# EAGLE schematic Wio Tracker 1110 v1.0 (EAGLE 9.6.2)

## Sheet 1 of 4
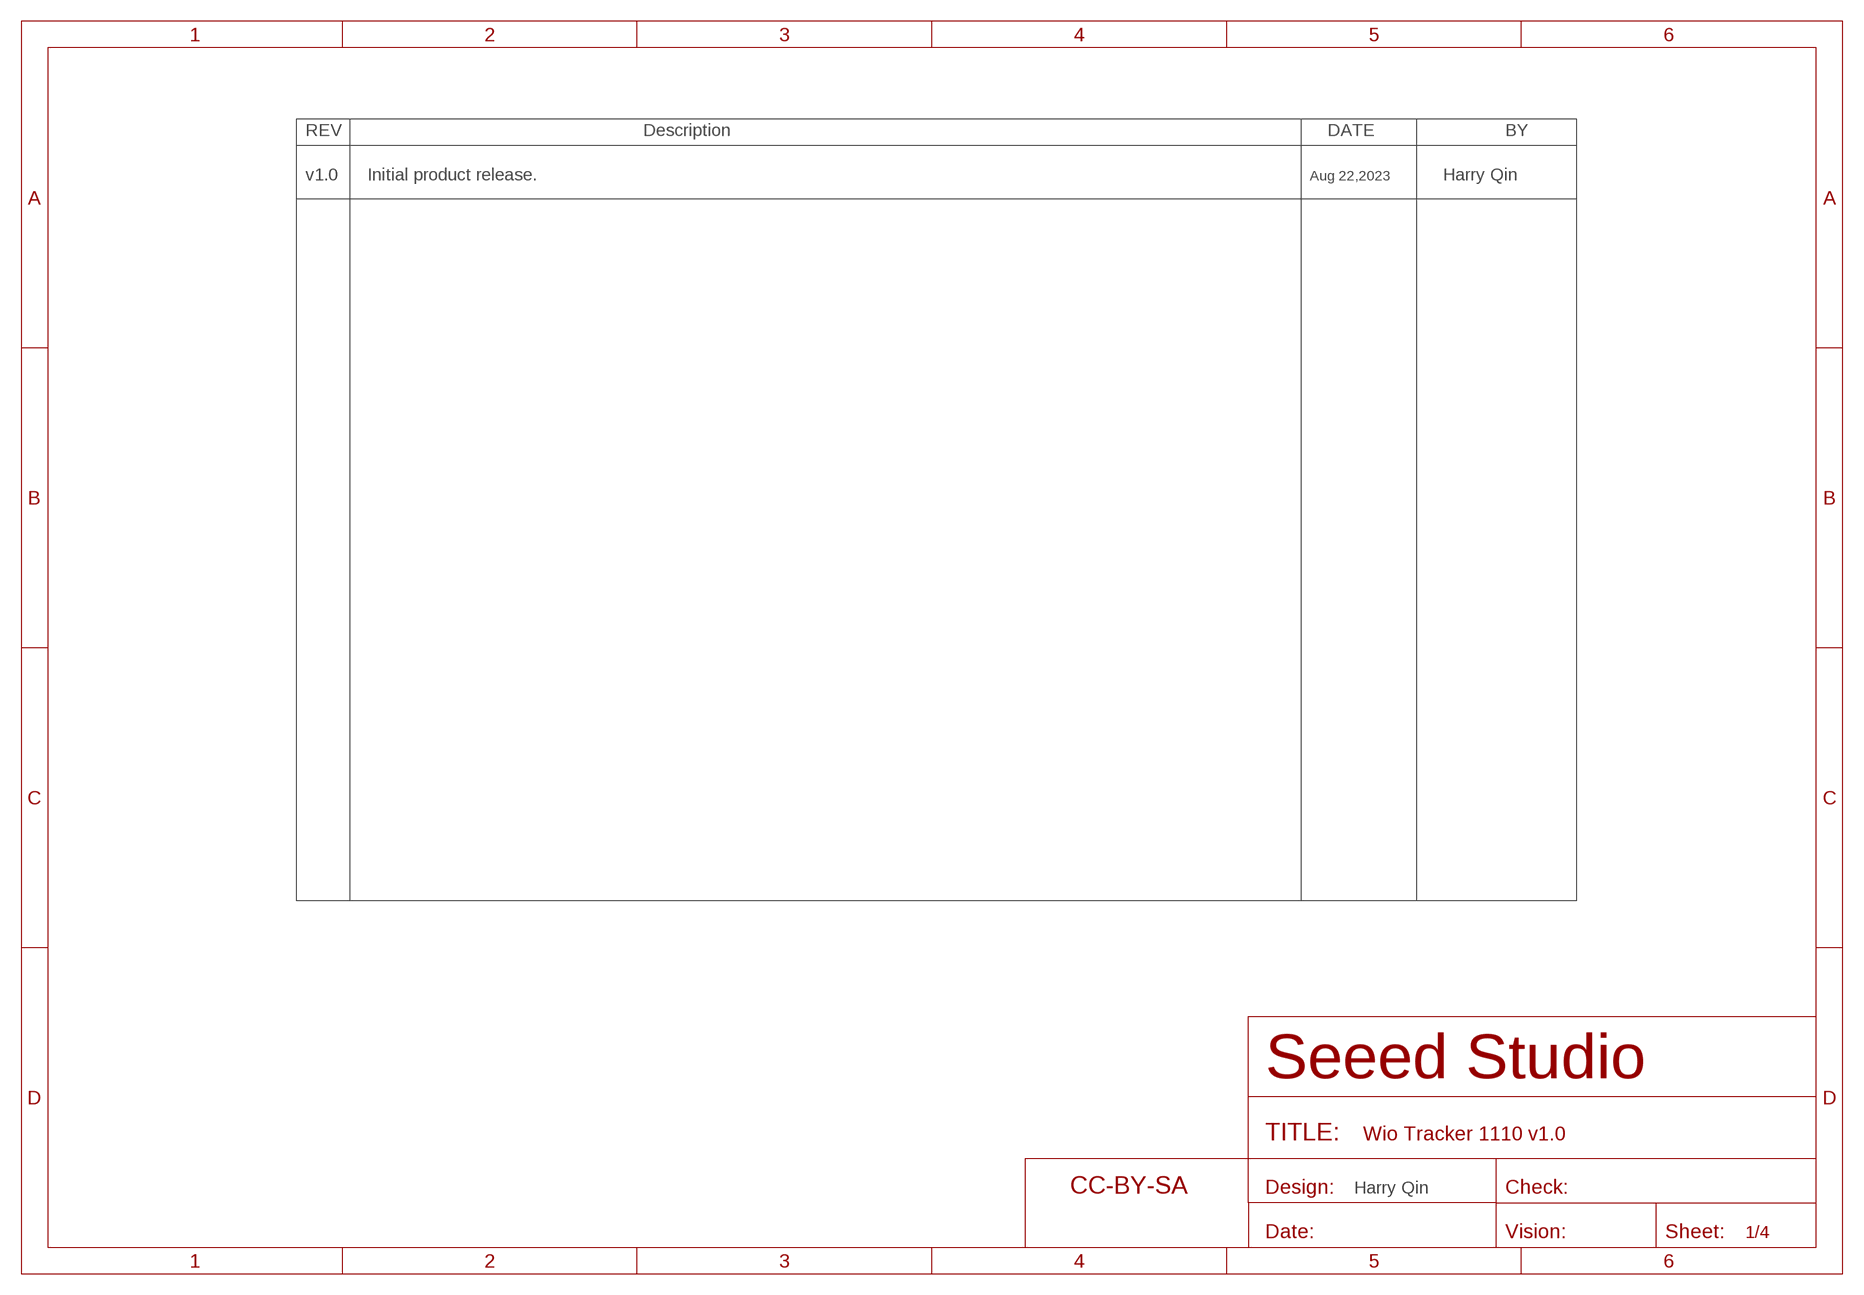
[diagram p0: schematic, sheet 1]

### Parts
FR2  SEEEDSTUDIO-OPEN-SCH-FRAME  [SEEEDSTUDIO-PCB-FRAME]

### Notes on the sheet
- v1.0 | Initial product release. | Aug 22,2023 | Harry Qin
- Harry Qin

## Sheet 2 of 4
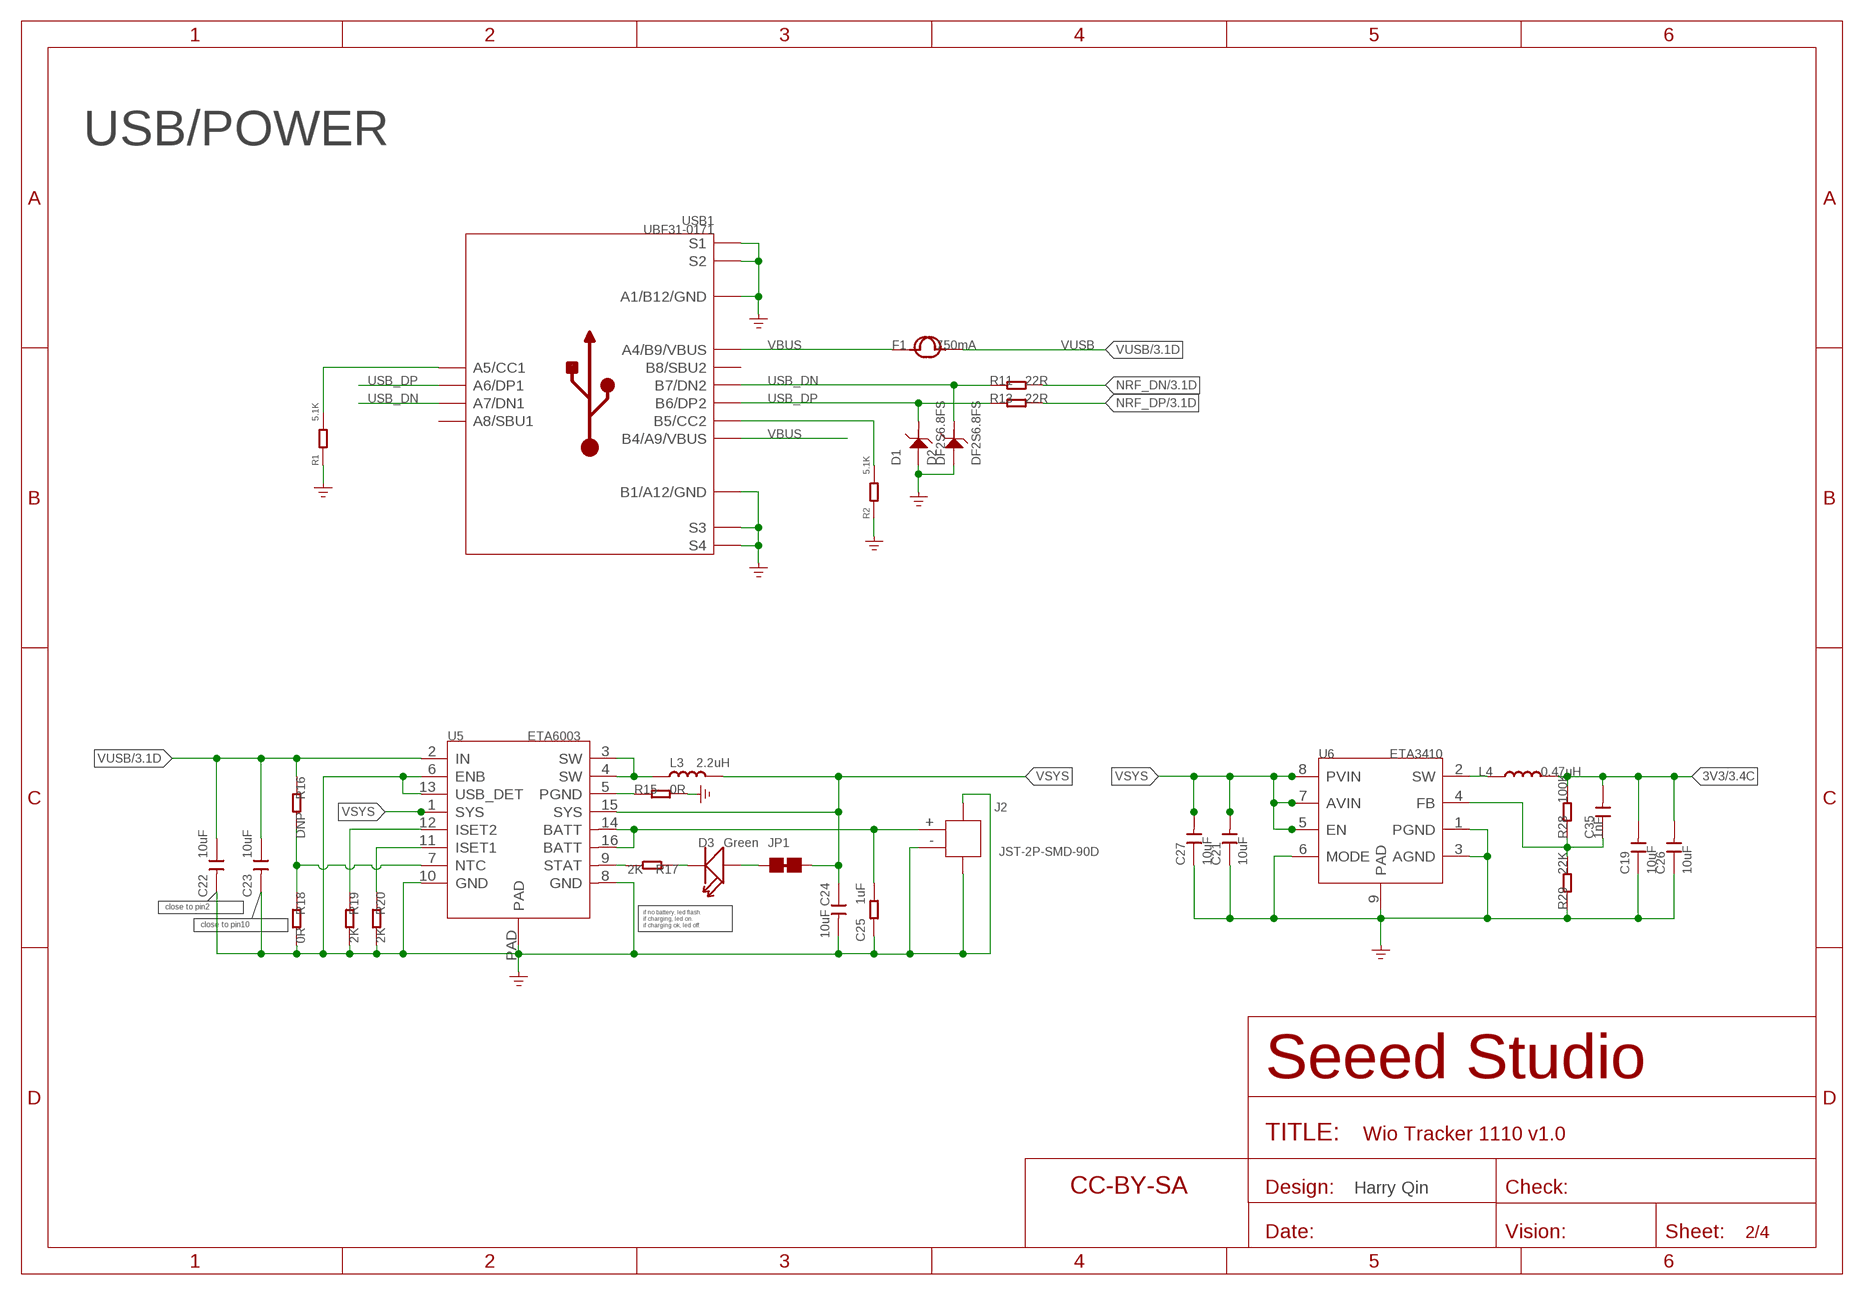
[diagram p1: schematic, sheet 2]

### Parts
C19  10uF  CAP-0603  [C0603]
C21  10uF  CAP-0603  [C0603]
C22  10uF  CAP-0805  [C0805]
C23  10uF  CAP-0805  [C0805]
C24  10uF  CAP-0805  [C0805]
C25  1uF  RES-0402  [R0402]
C26  10uF  CAP-0603  [C0603]
C27  10uF  CAP-0603  [C0603]
C35  1nF  CAP-0402  [C0402]
D1  DF2S6.8FS  D-ESD-2P'DF2S6.8FS'  [SOD-923]
D2  DF2S6.8FS  D-ESD-2P'DF2S6.8FS'  [SOD-923]
D3  Green  LED-0402  [LED-0402]
F1  750mA  FUSE+'1206'  [FS1206]
FR1  SEEEDSTUDIO-OPEN-SCH-FRAME  [SEEEDSTUDIO-PCB-FRAME]
J2  JST-2P-SMD-90D  JST-2P-SMD'2.0'  [HW2-SMD-2.0-90D]
JP1  JP-2P-SHORT'1'  [2P-SMD-SHORT]
L3  2.2uH  INDUCTOR'0806'  [L0806]
L4  0.47uH  L-MPM201610SR33_T  [L201610@1]
R1  5.1K  RES-0402  [R0402]
R2  5.1K  RES-0402  [R0402]
R11  22R  RES-0402  [R0402]
R13  22R  RES-0402  [R0402]
R15  0R  RES-0402  [R0402]
R16  DNP  RES-0402  [R0402]
R17  2K  RES-0402  [R0402]
R18  0R  RES-0402  [R0402]
R19  2K  RES-0402  [R0402]
R20  2K  RES-0402  [R0402]
R28  100K  RES-0402  [R0402]
R29  22K  RES-0402  [R0402]
U5  ETA6003  PMIC-ETA6003  [QFN16G-0.5-3X3MM]
U6  ETA3410  CONVERTER-ETA3410  [DFN8G-0.5-2X2MM]
USB1  UBF31-0171  USB2.0-TYPE-C-320010698  [USB2.0-TYPE-C]

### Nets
3V3: C19.2 C26.2 C35.2 L4.2 R28.2 ; also sheet 3,4
GND: C19.1 C21.1 C22.2 C23.2 C24.2 C25.2 C26.1 C27.1 D1.2 D2.2 J2.3 J2.4 J2.- R1.1 R2.1 R15.2 R18.2 R19.2 R20.2 R29.1 U5.6(ENB) U5.8(GND) U5.10(GND) U5.13(USB_DET) U5.PAD U6.1(PGND) U6.3(AGND) U6.6(MODE) U6.9(PAD) USB1.A1_B12(A1/B12/GND) USB1.B1_A12(B1/A12/GND) USB1.S1 USB1.S2 USB1.S3 USB1.S4 USB1.S5(S1) USB1.S6(S2) ; supply symbol labelled GND_POWER ; also sheet 3,4
N$1: R1.2 USB1.A5(A5/CC1)
N$2: R2.2 USB1.B5(B5/CC2)
N$10: D3.+ JP1.1
N$26: L3.1 U5.3(SW) U5.4(SW)
N$28: C25.1 J2.+ U5.14(BATT) U5.16(BATT)
N$29: L4.1 U6.2(SW)
N$30: D3.- R17.1
N$31: R17.2 U5.9(STAT)
N$32: C35.1 R28.1 R29.2 U6.4(FB)
N$33: R16.2 R18.1 U5.7(NTC)
N$34: R20.1 U5.11(ISET1)
N$36: R19.1 U5.12(ISET2)
N$37: R15.1 U5.5(PGND)
NRF_DN: R11.2 ; also sheet 3
NRF_DP: R13.2 ; also sheet 3
USB_DN: D2.1 R11.1 USB1.A7(A7/DN1) USB1.B7(B7/DN2)
USB_DP: D1.1 R13.1 USB1.A6(A6/DP1) USB1.B6(B6/DP2)
VBUS: F1.1 USB1.A4_B9(A4/B9/VBUS) USB1.B4_A9(B4/A9/VBUS)
VSYS: C21.2 C24.1 C27.2 JP1.2 L3.2 U5.1(SYS) U5.15(SYS) U6.5(EN) U6.7(AVIN) U6.8(PVIN)
VUSB: C22.1 C23.1 F1.2 R16.1 U5.2(IN) ; also sheet 3
Unconnected: USB1.A8(A8/SBU1) USB1.B8(B8/SBU2)

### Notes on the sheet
- USB/POWER
- close to pin2
- close to pin10
- if no battery, led flash.
  if charging, led on.
  if charging ok, led off.
- Harry Qin

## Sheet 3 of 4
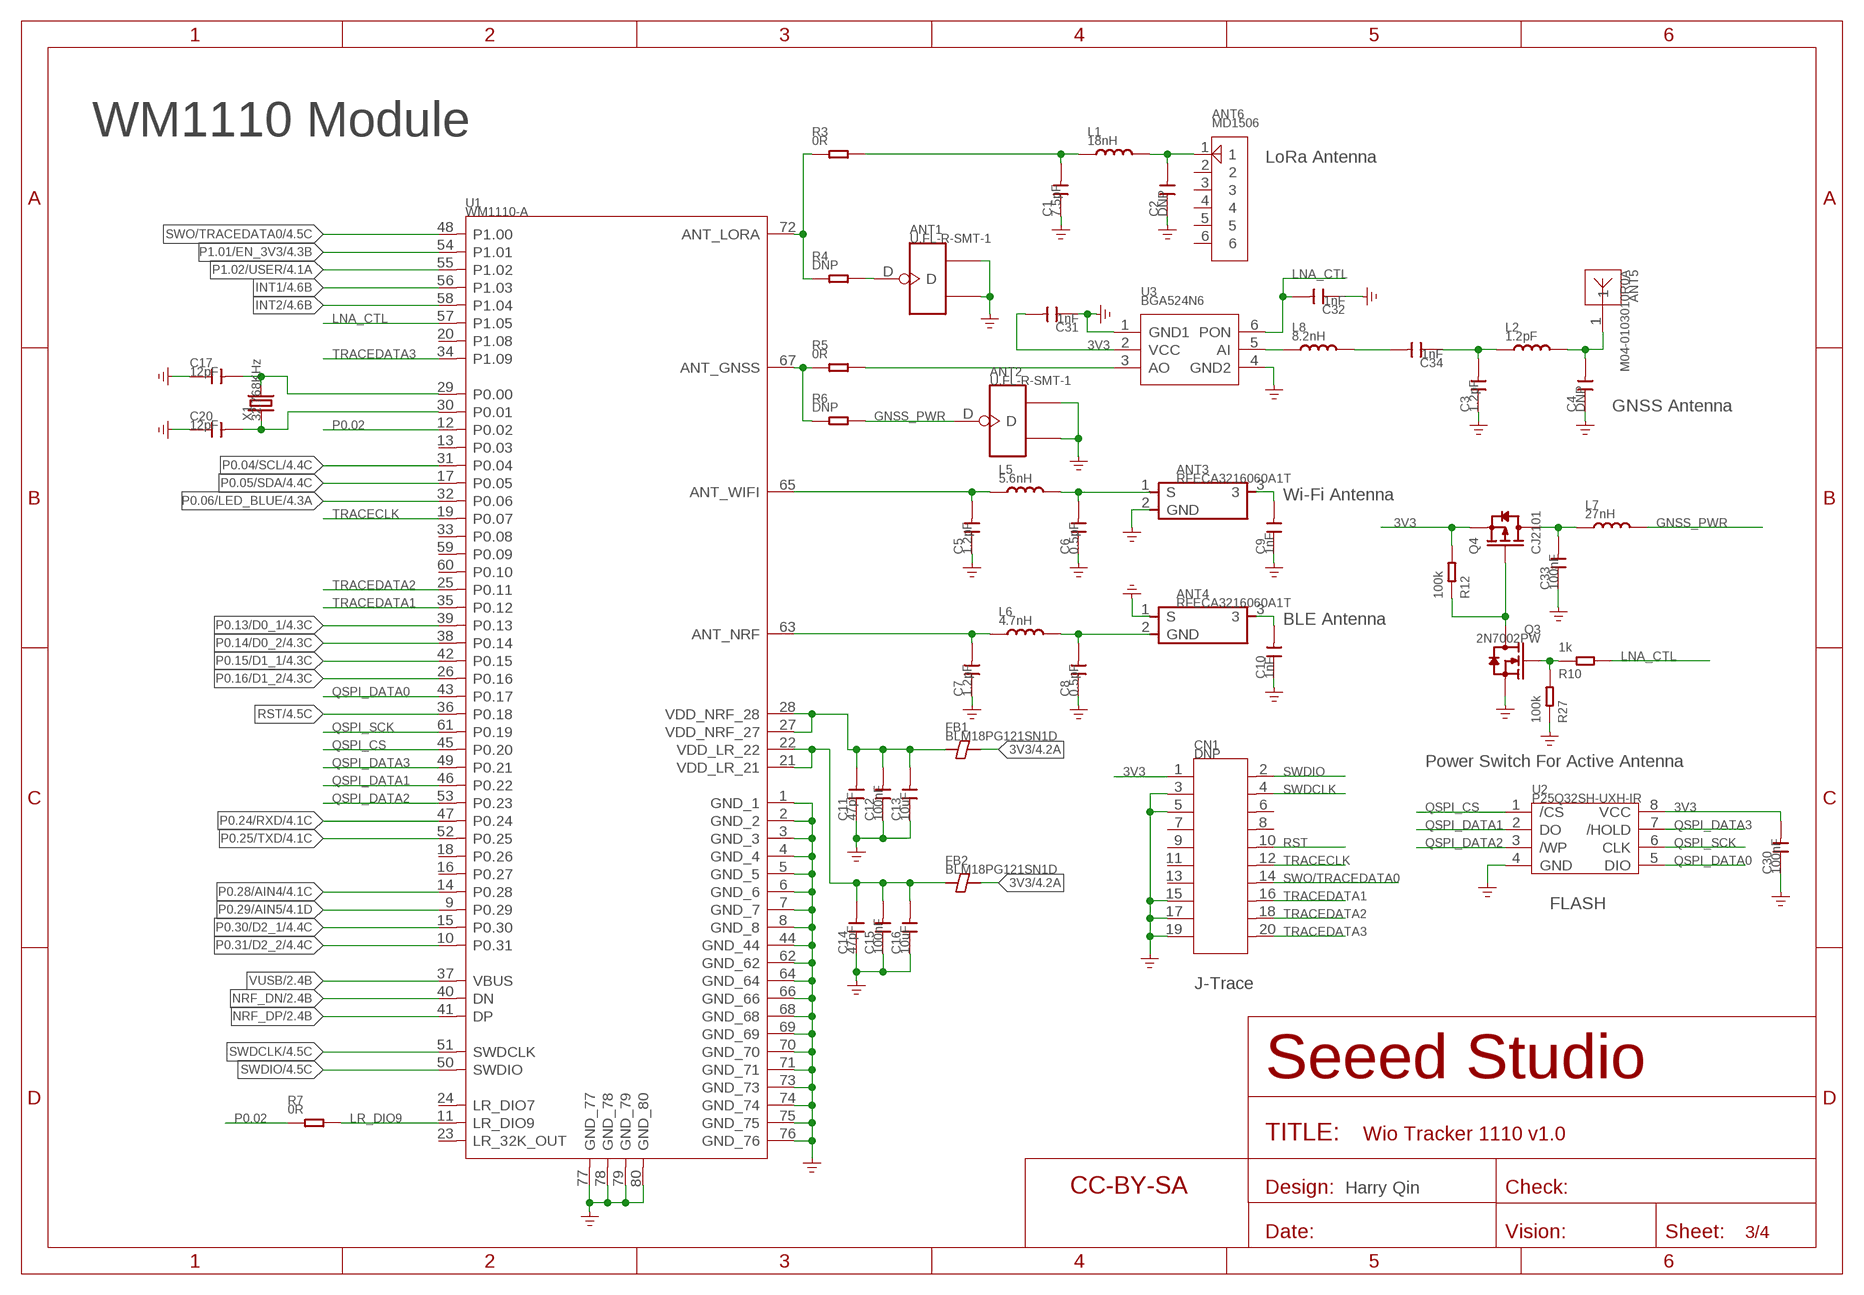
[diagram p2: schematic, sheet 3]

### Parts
ANT1  U.FL-R-SMT-1  ANTENNA-U-FL-320110048  [U-FL3P-SMD-2.6X2.6X1.0MM]
ANT2  U.FL-R-SMT-1  ANTENNA-U-FL-320110048  [U-FL3P-SMD-2.6X2.6X1.0MM]
ANT3  RFECA3216060A1T  ANTENNA-AN3116  [ANT-SMD3P-3.1X1.6X1.04MM]
ANT4  RFECA3216060A1T  ANTENNA-AN3116  [ANT-SMD3P-3.1X1.6X1.04MM]
ANT5  M04-0103010R0A  ANTENNA-M04-0103010R0A  [ANT-DIP-14X6X4MM]
ANT6  MD1506  ANTENNA-MD1506-12N  [ANT6-SMD-15X6.5X1.63MM]
C1  7.5pF  CAP-0402  [C0402]
C2  DNP  CAP-0402  [C0402]
C3  1.2pF  CAP-0402  [C0402]
C4  DNP  CAP-0402  [C0402]
C5  1.2pF  CAP-0402  [C0402]
C6  0.5pF  CAP-0402  [C0402]
C7  1.2pF  CAP-0402  [C0402]
C8  0.5pF  CAP-0402  [C0402]
C9  1nF  CAP-0402  [C0402]
C10  1nF  CAP-0402  [C0402]
C11  47pF  CAP-0402  [C0402]
C12  100nF  CAP-0402  [C0402]
C13  10uF  CAP-0603  [C0603]
C14  47pF  CAP-0402  [C0402]
C15  100nF  CAP-0402  [C0402]
C16  10uF  CAP-0603  [C0603]
C17  12pF  CAP-0402  [C0402]
C20  12pF  CAP-0402  [C0402]
C30  100nF  CAP-0402  [C0402]
C31  1nF  CAP-0402  [C0402]
C32  1nF  CAP-0402  [C0402]
C33  100nF  CAP-0402  [C0402]
C34  1nF  CAP-0402  [C0402]
CN1  DNP  HEADER-2X10P-1/3-1.27  [H2X10-1.27-12.7X3X5.7MM]
FB1  BLM18PG121SN1D  FERRITE-BEAD-0603  [F0603]
FB2  BLM18PG121SN1D  FERRITE-BEAD-0603  [F0603]
FR3  SEEEDSTUDIO-OPEN-SCH-FRAME  [SEEEDSTUDIO-PCB-FRAME]
L1  18nH  INDUCTOR'0402'  [L0402]
L2  1.2pF  INDUCTOR'0402'  [L0402]
L5  5.6nH  INDUCTOR'0402'  [L0402]
L6  4.7nH  INDUCTOR'0402'  [L0402]
L7  27nH  INDUCTOR'0402'  [L0402]
L8  8.2nH  INDUCTOR'0402'  [L0402]
Q3  2N7002PW  MOSFET-N-SI1304BDL  [SOT-323]
Q4  CJ2101  MOSFET-P-SOT323  [SOT-323]
R3  0R  RES-0402  [R0402]
R4  DNP  RES-0402  [R0402]
R5  0R  RES-0402  [R0402]
R6  DNP  RES-0402  [R0402]
R7  0R  RES-0402  [R0402]
R10  1k  RES-0402  [R0402]
R12  100k  RES-0402  [R0402]
R27  100k  RES-0402  [R0402]
U1  WM1110-A  MODULE-LORAMODULE  [MODULE72_0D9_20X20X2MM]
U2  P25Q32SH-UXH-IR  FLASH-W25X80-FZUIH1  [USON8-0.5-3X2MM]
U3  BGA524N6  GNSS-BGA524N6  [BGA6-0.4-1.1X0.7X0.4MM]
X1  32.768KHz  CRYSTAL-2P'NX2012SA'  [X2-SMD-L2.0X1.2X0.55MM]

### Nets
3V3: C30.2 C31.2 CN1.1 FB1.2 FB2.2 Q4.2(S) R12.2 U2.8(VCC) U3.2(VCC) ; also sheet 2,4
GND: ANT1.GND1 ANT1.GND2 ANT2.GND1 ANT2.GND2 ANT3.2(GND) ANT4.1(S) C1.1 C2.1 C3.1 C4.1 C5.1 C6.1 C7.1 C8.1 C9.1 C10.1 C11.1 C12.1 C13.1 C14.1 C15.1 C16.1 C17.1 C20.1 C30.1 C31.1 C32.1 C33.1 CN1.3 CN1.5 CN1.15 CN1.17 CN1.19 Q3.2(S) R27.1 U1.1(GND_1) U1.2(GND_2) U1.3(GND_3) U1.4(GND_4) U1.5(GND_5) U1.6(GND_6) U1.7(GND_7) U1.8(GND_8) U1.44(GND_44) U1.62(GND_62) U1.64(GND_64) U1.66(GND_66) U1.68(GND_68) U1.69(GND_69) U1.70(GND_70) U1.71(GND_71) U1.73(GND_73) U1.74(GND_74) U1.75(GND_75) U1.76(GND_76) U1.77(GND_77) U1.78(GND_78) U1.79(GND_79) U1.80(GND_80) U2.4(GND) U3.1(GND1) U3.4(GND2) ; supply symbol labelled GND_POWER ; also sheet 2,4
GNSS_PWR: ANT2.D L7.2 R6.2
INT1: U1.56(P1.03) ; also sheet 4
INT2: U1.58(P1.04) ; also sheet 4
LNA_CTL: C32.2 R10.2 U1.57(P1.05) U3.6(PON)
LR_DIO9: R7.2 U1.11(LR_DIO9)
N$3: C1.2 L1.1 R3.2
N$4: ANT6.1 C2.2 L1.2
N$5: R3.1 R4.1 U1.72(ANT_LORA)
N$6: C3.2 C34.1 L2.1
N$8: Q3.3(D) Q4.1(G) R12.1
N$9: Q3.1(G) R10.1 R27.2
N$12: C5.2 L5.1 U1.65(ANT_WIFI)
N$13: C17.2 U1.29(P0.00) X1.2
N$15: ANT3.1(S) C6.2 L5.2
N$16: C7.2 L6.1 U1.63(ANT_NRF)
N$17: C20.2 U1.30(P0.01) X1.1
N$18: ANT4.2(GND) C8.2 L6.2
N$19: ANT3.3 C9.2
N$20: ANT4.3 C10.2
N$21: ANT1.D R4.2
N$23: ANT5.1 C4.2 L2.2
N$24: R5.2 U3.3(AO)
N$25: R5.1 R6.1 U1.67(ANT_GNSS)
N$27: C33.2 L7.1 Q4.3(D)
N$35: L8.1 U3.5(AI)
N$42: C34.2 L8.2
NRF_DN: U1.40(DN) ; also sheet 2
NRF_DP: U1.41(DP) ; also sheet 2
P0.02: R7.1 U1.12(P0.02)
P0.04/SCL: U1.31(P0.04) ; also sheet 4
P0.05/SDA: U1.17(P0.05) ; also sheet 4
P0.06/LED_BLUE: U1.32(P0.06) ; also sheet 4
P0.13/D0_1: U1.39(P0.13) ; also sheet 4
P0.14/D0_2: U1.38(P0.14) ; also sheet 4
P0.15/D1_1: U1.42(P0.15) ; also sheet 4
P0.16/D1_2: U1.26(P0.16) ; also sheet 4
P0.24/RXD: U1.47(P0.24) ; also sheet 4
P0.25/TXD: U1.52(P0.25) ; also sheet 4
P0.28/AIN4: U1.14(P0.28) ; also sheet 4
P0.29/AIN5: U1.9(P0.29) ; also sheet 4
P0.30/D2_1: U1.15(P0.30) ; also sheet 4
P0.31/D2_2: U1.10(P0.31) ; also sheet 4
P1.01/EN_3V3: U1.54(P1.01) ; also sheet 4
P1.02/USER: U1.55(P1.02) ; also sheet 4
QSPI_CS: U1.45(P0.20) U2.1(/CS)
QSPI_DATA0: U1.43(P0.17) U2.5(DIO)
QSPI_DATA1: U1.46(P0.22) U2.2(DO)
QSPI_DATA2: U1.53(P0.23) U2.3(/WP)
QSPI_DATA3: U1.49(P0.21) U2.7(/HOLD)
QSPI_SCK: U1.61(P0.19) U2.6(CLK)
RST: CN1.10 U1.36(P0.18) ; also sheet 4
SWDCLK: CN1.4 U1.51(SWDCLK) ; also sheet 4
SWDIO: CN1.2 U1.50(SWDIO) ; also sheet 4
SWO/TRACEDATA0: CN1.14 U1.48(P1.00) ; also sheet 4
TRACECLK: CN1.12 U1.19(P0.07)
TRACEDATA1: CN1.16 U1.35(P0.12)
TRACEDATA2: CN1.18 U1.25(P0.11)
TRACEDATA3: CN1.20 U1.34(P1.09)
VDD_LR: C14.2 C15.2 C16.2 FB2.1 U1.21(VDD_LR_21) U1.22(VDD_LR_22)
VDD_NRF: C11.2 C12.2 C13.2 FB1.1 U1.27(VDD_NRF_27) U1.28(VDD_NRF_28)
VUSB: U1.37(VBUS) ; also sheet 2
Unconnected: ANT6.2 ANT6.3 ANT6.4 ANT6.5 ANT6.6 CN1.6 CN1.7 CN1.8 CN1.9 CN1.11 CN1.13 U1.13(P0.03) U1.16(P0.27) U1.18(P0.26) U1.20(P1.08) U1.23(LR_32K_OUT) U1.24(LR_DIO7) U1.33(P0.08) U1.59(P0.09) U1.60(P0.10)

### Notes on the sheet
- WM1110 Module
- LoRa Antenna
- GNSS Antenna
- Wi-Fi Antenna
- BLE Antenna
- Power Switch For Active Antenna
- FLASH
- J-Trace
- Harry Qin

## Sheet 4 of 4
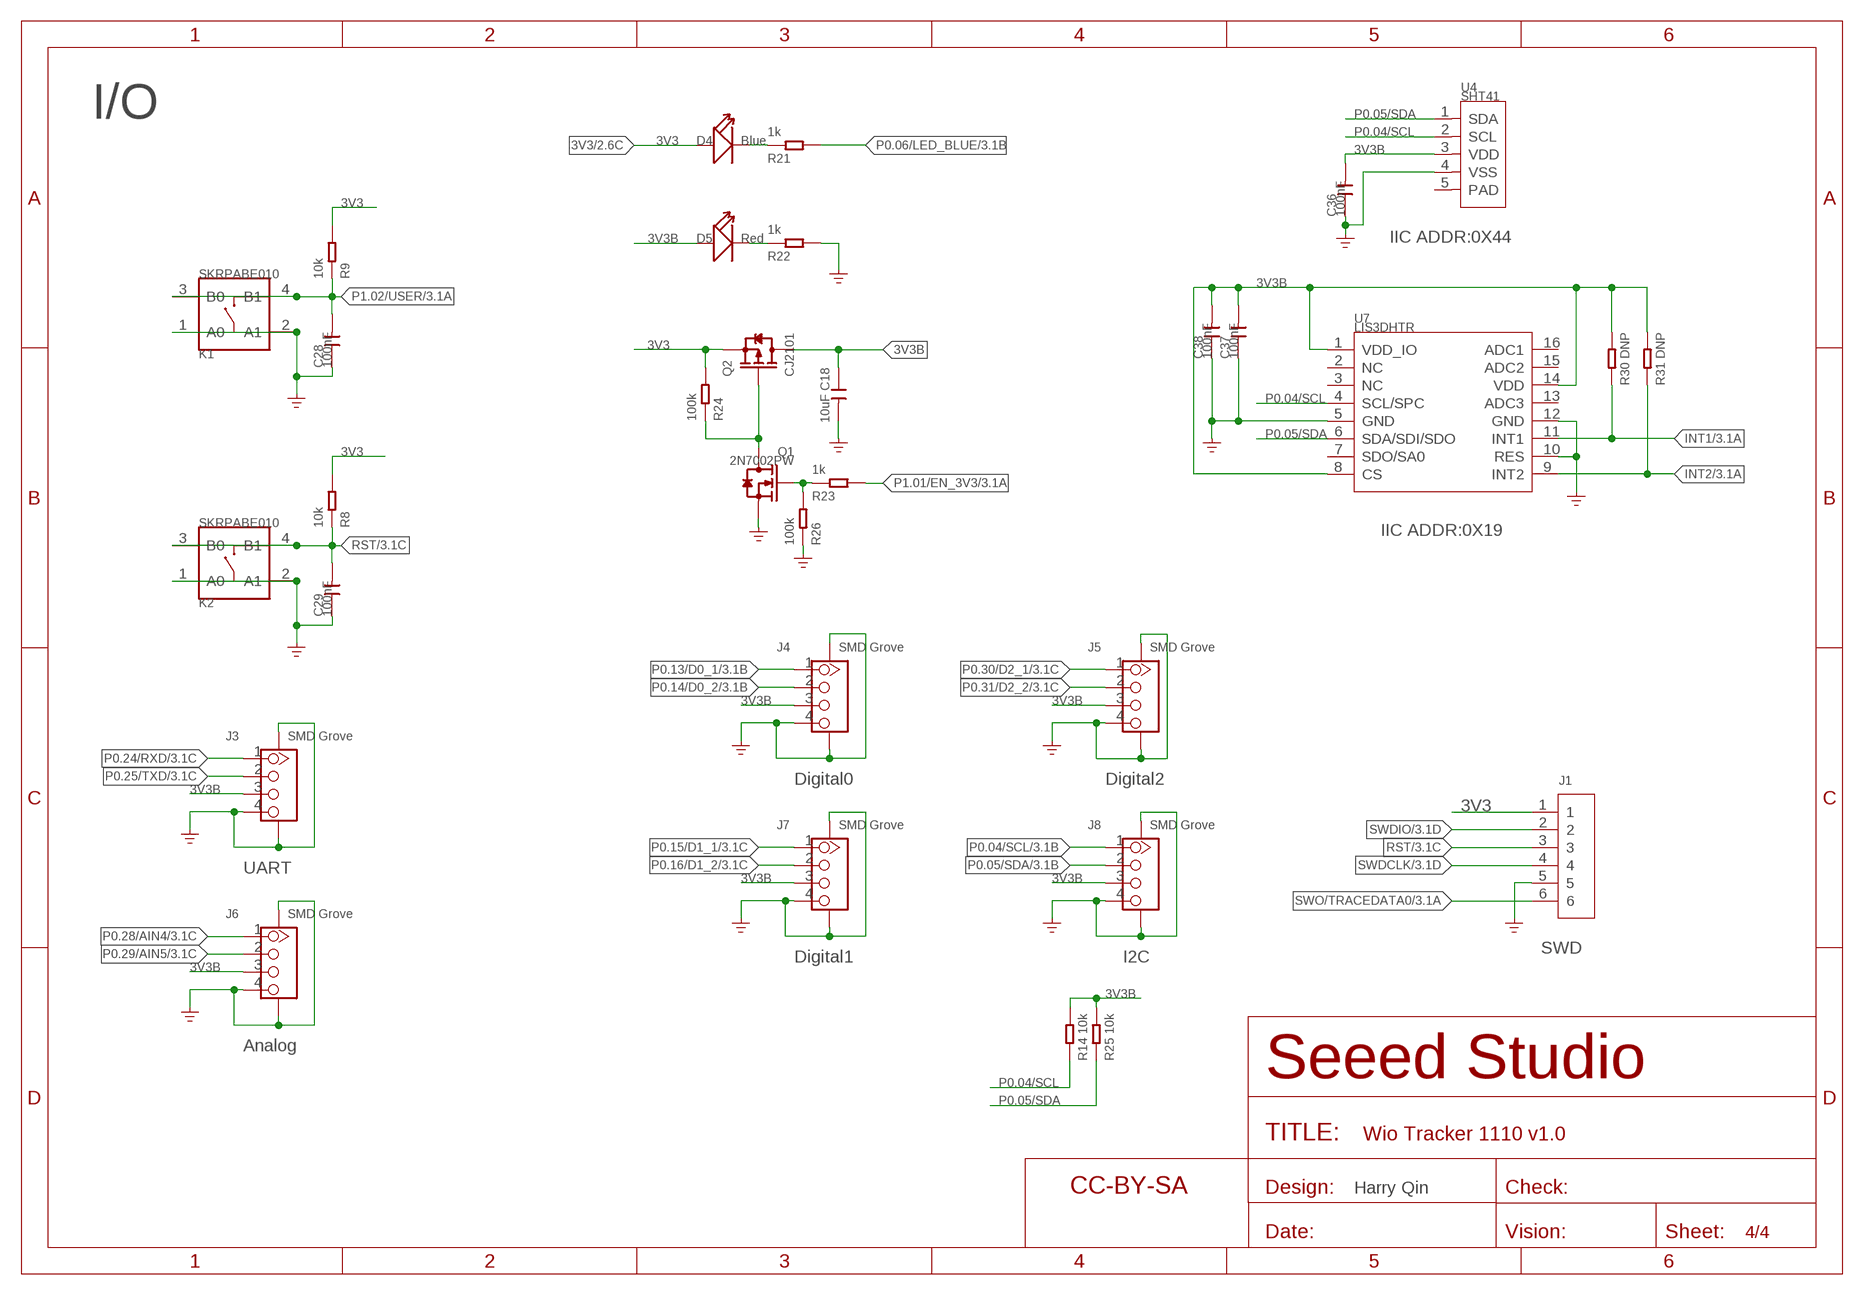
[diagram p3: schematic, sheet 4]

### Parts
C18  10uF  CAP-0805  [C0805]
C28  100nF  CAP-0402  [C0402]
C29  100nF  CAP-0402  [C0402]
C36  100nF  CAP-0402  [C0402]
C37  100nF  CAP-0402  [C0402]
C38  100nF  CAP-0402  [C0402]
D4  Blue  LED'0603'  [LED-0603]
D5  Red  LED'0603'  [LED-0603]
FR4  SEEEDSTUDIO-OPEN-SCH-FRAME  [SEEEDSTUDIO-PCB-FRAME]
J1  CONNECTOR-TC2030-IDC-NL  [CONNECTER6P-1.27-9.9X6.1MM]
J3  SMD Grove  GROVE-CONNECTOR-SMD'90D'  [HW4-SMD-2.0-90D]
J4  SMD Grove  GROVE-CONNECTOR-SMD'90D'  [HW4-SMD-2.0-90D]
J5  SMD Grove  GROVE-CONNECTOR-SMD'90D'  [HW4-SMD-2.0-90D]
J6  SMD Grove  GROVE-CONNECTOR-SMD'90D'  [HW4-SMD-2.0-90D]
J7  SMD Grove  GROVE-CONNECTOR-SMD'90D'  [HW4-SMD-2.0-90D]
J8  SMD Grove  GROVE-CONNECTOR-SMD'90D'  [HW4-SMD-2.0-90D]
K1  SKRPABE010  BUTTON-4P-4.5X3.2  [SW4P-SMD-4.5X3.2X2.5MM]
K2  SKRPABE010  BUTTON-4P-4.5X3.2  [SW4P-SMD-4.5X3.2X2.5MM]
Q1  2N7002PW  MOSFET-N-SI1304BDL  [SOT-323]
Q2  CJ2101  MOSFET-P-SOT323  [SOT-323]
R8  10k  RES-0402  [R0402]
R9  10k  RES-0402  [R0402]
R14  10k  RES-0402  [R0402]
R21  1k  RES-0402  [R0402]
R22  1k  RES-0402  [R0402]
R23  1k  RES-0402  [R0402]
R24  100k  RES-0402  [R0402]
R25  10k  RES-0402  [R0402]
R26  100k  RES-0402  [R0402]
R30  DNP  RES-0402  [R0402]
R31  DNP  RES-0402  [R0402]
U4  SHT41  SENSOR-SHT40  [SNR4-0.8-1.5X1.5X0.54MM]
U7  LIS3DHTR  SENSOR-MOTION/POSITION-LIS3DH-314080105  [LGA16-0.5-3X3MM]

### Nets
3V3: D4.+ J1.1 Q2.2(S) R8.2 R9.2 R24.2 ; also sheet 2,3
3V3B: C18.1 C36.2 C37.2 C38.2 D5.+ J3.3 J4.3 J5.3 J6.3 J7.3 J8.3 Q2.3(D) R14.2 R25.2 R30.2 R31.2 U4.3(VDD) U7.1(VDD_IO) U7.8(CS) U7.14(VDD)
GND: C18.2 C28.1 C29.1 C36.1 C37.1 C38.1 J1.5 J3.4 J3.SS1 J3.SS2 J4.4 J4.SS1 J4.SS2 J5.4 J5.SS1 J5.SS2 J6.4 J6.SS1 J6.SS2 J7.4 J7.SS1 J7.SS2 J8.4 J8.SS1 J8.SS2 K1.1(A0) K1.2(A1) K2.1(A0) K2.2(A1) Q1.2(S) R22.2 R26.1 U4.4(VSS) U7.5(GND) U7.10(RES) U7.12(GND) ; supply symbol labelled GND_POWER ; also sheet 2,3
INT1: R30.1 U7.11(INT1) ; also sheet 3
INT2: R31.1 U7.9(INT2) ; also sheet 3
N$7: Q1.3(D) Q2.1(G) R24.1
N$11: Q1.1(G) R23.1 R26.2
N$14: D4.- R21.1
N$22: D5.- R22.1
P0.04/SCL: J8.1 R14.1 U4.2(SCL) U7.4(SCL/SPC) ; also sheet 3
P0.05/SDA: J8.2 R25.1 U4.1(SDA) U7.6(SDA/SDI/SDO) ; also sheet 3
P0.06/LED_BLUE: R21.2 ; also sheet 3
P0.13/D0_1: J4.1 ; also sheet 3
P0.14/D0_2: J4.2 ; also sheet 3
P0.15/D1_1: J7.1 ; also sheet 3
P0.16/D1_2: J7.2 ; also sheet 3
P0.24/RXD: J3.1 ; also sheet 3
P0.25/TXD: J3.2 ; also sheet 3
P0.28/AIN4: J6.1 ; also sheet 3
P0.29/AIN5: J6.2 ; also sheet 3
P0.30/D2_1: J5.1 ; also sheet 3
P0.31/D2_2: J5.2 ; also sheet 3
P1.01/EN_3V3: R23.2 ; also sheet 3
P1.02/USER: C28.2 K1.3(B0) K1.4(B1) R9.1 ; also sheet 3
RST: C29.2 J1.3 K2.3(B0) K2.4(B1) R8.1 ; also sheet 3
SWDCLK: J1.4 ; also sheet 3
SWDIO: J1.2 ; also sheet 3
SWO/TRACEDATA0: J1.6 ; also sheet 3
Unconnected: U4.5(PAD) U7.2(NC) U7.3(NC) U7.7(SDO/SA0) U7.13(ADC3) U7.15(ADC2) U7.16(ADC1)

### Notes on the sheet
- I/O
- IIC ADDR:0X44
- IIC ADDR:0X19
- Digital0 | Digital2
- UART
- SWD
- Digital1 | I2C
- Analog
- Harry Qin

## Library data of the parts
ANT1 ANT2 = Connector-new:ANTENNA-U-FL
ANT3 ANT4 = Connector-new:ANTENNA-AN3116
ANT5 = Connector-new:ANTENNA-M04-0103010R0A
ANT6 = Connector-new:ANTENNA-MD1506-12N
C1-C24 C26-C38 = Discrete-new:CAP: Ceramic Capacitors
C25 R1-R31 = Discrete-new:RES
CN1 = Connector-new:HEADER-2X10P-1/3
D1 D2 = Discrete-new:D-ESD-2P: SOD-923:304060009;SOD-123:304060001
D3-D5 = Discrete-new:LED
F1 = Discrete-new:FUSE+
FB1 FB2 = Discrete-new:FERRITE-BEAD
FR1-FR4 = moudle-new:SEEEDSTUDIO-OPEN-SCH-FRAME
J1 = Connector-new:CONNECTOR-TC2030-IDC-NL
J2 = Connector-new:JST-2P-SMD: 2P-SMD-1.0-90D:320110054;2P-SMD-2.0-90D:320110026
J3-J8 = Connector-new:GROVE-CONNECTOR-SMD: 4P-SMD-2.0:320110030;4P-SMD-2.0-90D:320110032
JP1 = Discrete-new:JP-2P-SHORT
K1 K2 = Discrete-new:BUTTON-4P: SW4-6.0X6.0X5.0MM:311020024;SW4-8.0X8.0X9.0MM:311020028;SW4-SMD-6.0X6.0X5.0MM:311020004;SW4-SMD-3.35X3.35X1.5MM:311020030;SW4-SMD-5.2X5.2X2.5MM:311020046
L1-L3 L5-L8 = Discrete-new:INDUCTOR
L4 = Discrete-new:L
Q1 Q3 = Discrete-new:MOSFET-N: IRLL014: http://www.vishay.com/docs/91319/sihll014.pdf
Q2 Q4 = Discrete-new:MOSFET-P
U1 = moudle-new:MODULE-LORAMODULE
U2 = IC-new:FLASH-W25X80: 1M-BIT,2M-BIT,4M-BIT AND 8M-BIT SERIAL FLASH MEMORY WITH 4KB SECTORS AND DUAL OUTPUT SPI
U3 = IC-new:GNSS-BGA524N6
U4 = Sensor:SENSOR-SHT40
U5 = template:PMIC-ETA6003: 2.5A,3MHZ Switching Charger with Dynamic Power Path Management
U6 = IC-new:CONVERTER-ETA3410: 3MHZ 2A High Step-Down Converter in DFN2x2-8L Package
U7 = Sensor:SENSOR-MOTION/POSITION-LIS3DH
USB1 = Connector-new:USB2.0-TYPE-C
X1 = Discrete-new:CRYSTAL-2P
